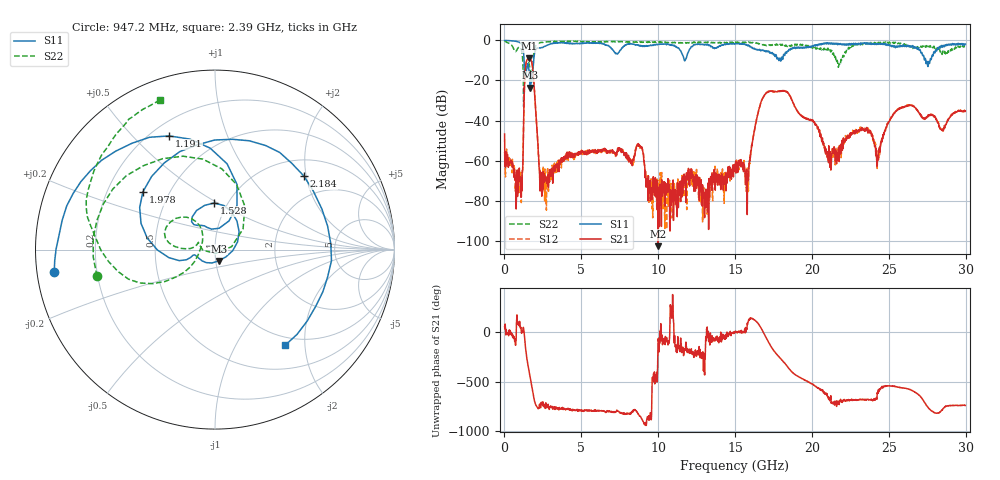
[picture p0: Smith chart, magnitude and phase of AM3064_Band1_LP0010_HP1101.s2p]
# Hz S DB R 50.0
!freq dBS11 angS11 dBS21 angS21 dBS12 angS12 dBS22 angS22
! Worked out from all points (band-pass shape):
!   1600 points, 10 MHz to 29.98 GHz, reference 50 ohm
!   highest |S21| = -8.87 dB at 1.622 GHz (marker M1); lowest = -102.6 dB at 10 GHz (marker M2)
!   |S21| within 3 dB of the highest: 1.392 GHz to 1.798 GHz (406 MHz wide, 25.4 % of centre)
!   lowest |S11| = -23.6 dB at 1.678 GHz (marker M3), VSWR 1.14, Z = 51.8 - j6.52 ohm
!   |S11| at or under -10 dB: 1.277 GHz to 1.902 GHz (625.2 MHz wide, 39.3 % of centre); 11.70538 GHz to 11.74881 GHz (43.43 MHz wide, 0.37 % of centre); 27.4 GHz to 27.68 GHz (282.6 MHz wide, 1.03 % of centre)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
!   |S22| runs from -33.0 to -0.3 dB; largest |S21 - S12| = 0.0054
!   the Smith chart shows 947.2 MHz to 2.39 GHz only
!   S11 on the Smith chart (normalised r, x): 947.2 MHz: 0.05, -0.07; 1.191 GHz: 0.27, +0.64; 1.528 GHz: 0.86, +0.48; 1.978 GHz: 0.36, +0.31; 2.184 GHz: 1.39, +1.94; 2.39 GHz: 0.87, -1.63
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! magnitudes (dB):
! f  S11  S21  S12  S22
! 10 MHz  -0.1  -46.8  -55.7  -0.3
! 947.2 MHz  -0.9  -67.2  -65.5  -3.4
! 1.191 GHz  -3.3  -64.4  -61.7  -10.7
! 1.528 GHz  -11.7  -9.2  -9.1  -10.5
! 1.622 GHz  -17.5  -8.9  -8.8  -12.4
! 1.678 GHz  -23.6  -9.1  -9.1  -16.0
! 1.978 GHz  -5.8  -28.4  -28.4  -3.9
! 2.184 GHz  -3.8  -52.5  -52.9  -1.6
! 2.39 GHz  -3.6  -66.0  -67.4  -1.0
! 5.015 GHz  -1.4  -54.7  -54.9  -0.8
! 8.782 GHz  -2.6  -52.7  -52.7  -0.9
! 10 GHz  -2.0  -102.6  -72.6  -0.9
! 13.04 GHz  -2.2  -77.0  -78.3  -1.1
! 15 GHz  -1.7  -62.9  -61.6  -1.3
! 15.81 GHz  -2.7  -71.1  -66.2  -1.2
! 17.14 GHz  -5.7  -25.6  -25.6  -2.7
! 19.99 GHz  -3.4  -40.0  -40.0  -3.4
! 21.15 GHz  -1.3  -57.4  -57.6  -4.3
! 23.29 GHz  -1.3  -44.6  -43.6  -2.2
! 24.3 GHz  -1.8  -57.7  -56.7  -1.1
! 25 GHz  -2.0  -40.9  -40.6  -1.2
! 29.98 GHz  -1.9  -35.3  -35.0  -3.2
